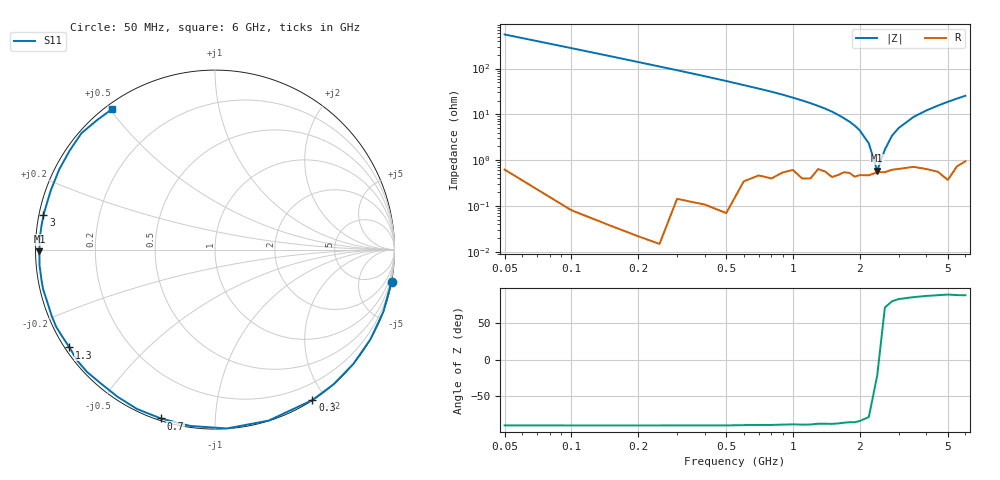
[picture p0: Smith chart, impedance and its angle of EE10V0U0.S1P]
! Infineon Technologies  Discrete & RF Semiconductors
! BBY55-02W
! Si Tuning Diode in SCD-80
! VR = 10 V
! S-Parameters:  June  2000
# GHz  S  MA  R  50
!  f  S11
! GHz  MAG  ANG
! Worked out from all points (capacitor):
!   34 points, 50 MHz to 6 GHz, reference 50 ohm
!   read as one part to ground: C = 5.69 pF near 50 MHz
!   lowest |Z| = 586 mohm at 2.4 GHz (marker M1)
!   series resonance near 2.424 GHz, so ESL is about 760 pH
!   S11 on the Smith chart (normalised r, x): 50 MHz: 0, -11; 300 MHz: 0.00, -1.84; 700 MHz: 0.01, -0.73; 1.3 GHz: 0.01, -0.30; 3 GHz: 0.01, +0.10; 6 GHz: 0.02, +0.51
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0.05  0.9998 -10.3
0.1  0.9999 -20.3
0.15  0.9999 -30.1
0.2  0.9999 -39.6
0.25  0.9999 -48.6
0.3  0.9987 -57.1
0.4  0.9985 -72.6
0.5  0.9987 -86.2
0.6  0.9922 -98.0
0.7  0.988 -107.8
0.8  0.9886 -116.1
0.9  0.9834 -123.6
1  0.9801 -130.4
1.1  0.9864 -136.2
1.2  0.9859 -141.4
1.3  0.9769 -146.1
1.5  0.9839 -154.2
1.6  0.9819 -158.0
1.7  0.9791 -161.4
1.9  0.983 -167.1
2.2  0.9816 -174.8
2.4  0.9785 -179.5
3  0.9749 168.6
3.5  0.9727 160.2
4  0.9762 152.7
5  0.9871 138.9
5.5  0.9758 132.3
6  0.9705 126.1
